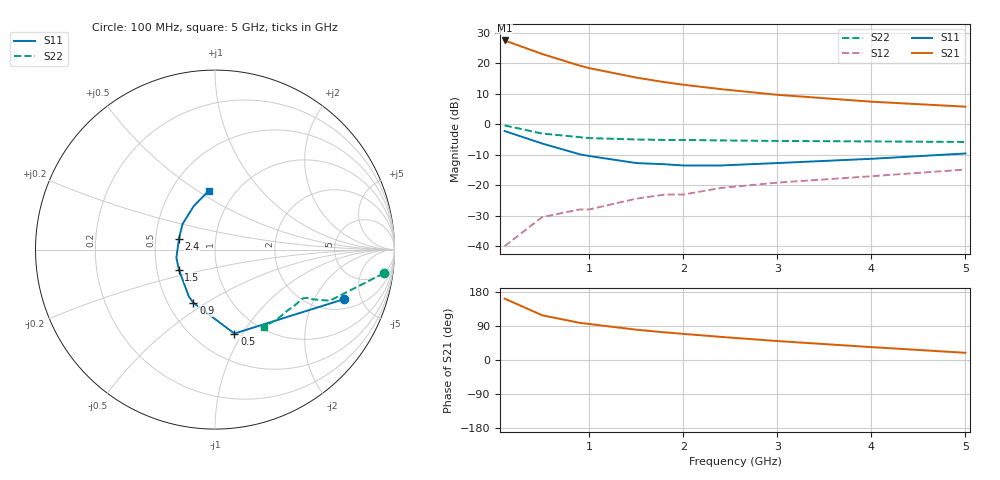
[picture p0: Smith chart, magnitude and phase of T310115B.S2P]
!AT-31011
!S and NOISE PARAMETERS at Vce=5V  Ic=10mA.  LAST UPDATED 04-10-94
# ghz s ma r 50
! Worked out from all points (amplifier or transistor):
!   11 points, 100 MHz to 5 GHz, reference 50 ohm
!   highest |S21| = 27.4 dB at 100 MHz (marker M1)
!   |S21| within 3 dB of that: start of sweep to 370.2 MHz
!   unconditionally stable (mu >= 1): 1.345 GHz to 4.721 GHz
!   at 500 MHz: K = 0.62, MSG = 26.7 dB, |S12| = -30.5 dB
!   at 1.8 GHz: K = 1.04, MAG = 17.2 dB, |S12| = -23.1 dB
!   at 5 GHz: K = 0.98, MSG = 10.3 dB, |S12| = -14.9 dB
!   lowest NFmin = 1.30 dB at 500 MHz
!   S11 on the Smith chart (normalised r, x): 100 MHz: 2.62, -3.56; 500 MHz: 0.76, -0.92; 900 MHz: 0.67, -0.44; 1.5 GHz: 0.65, -0.15; 2.4 GHz: 0.66, +0.08; 5 GHz: 0.76, +0.56
0.1  0.77 -21.0  23.46 162.0  0.01 80.0  0.95 -8.0
0.5  0.48 -77.0  14.07 118.0  0.03 61.0  0.7 -24.0
0.9  0.32 -112.0  9.06 98.0  0.04 59.0  0.61 -27.0
1  0.3 -119.0  8.26 95.0  0.04 60.0  0.59 -27.0
1.5  0.23 -151.0  5.78 80.0  0.06 60.0  0.56 -29.0
1.8  0.22 -168.0  4.87 73.0  0.07 60.0  0.55 -31.0
2  0.21 -178.0  4.42 69.0  0.07 60.0  0.55 -32.0
2.4  0.21 163.0  3.74 61.0  0.09 59.0  0.54 -36.0
3  0.23 142.0  3.02 50.0  0.11 58.0  0.53 -39.0
4  0.27 116.0  2.33 34.0  0.14 54.0  0.52 -48.0
5  0.33 96.0  1.93 19.0  0.18 48.0  0.51 -58.0
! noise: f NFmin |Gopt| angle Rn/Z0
0.5  1.3  0.45  11  0.55
0.9  1.4  0.37  33  0.46
1.8  1.7  0.25  86  0.29
2.4  2  0.18  129  0.18
